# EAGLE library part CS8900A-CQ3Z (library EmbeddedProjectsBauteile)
Crystal LAN - Ethernet Controller
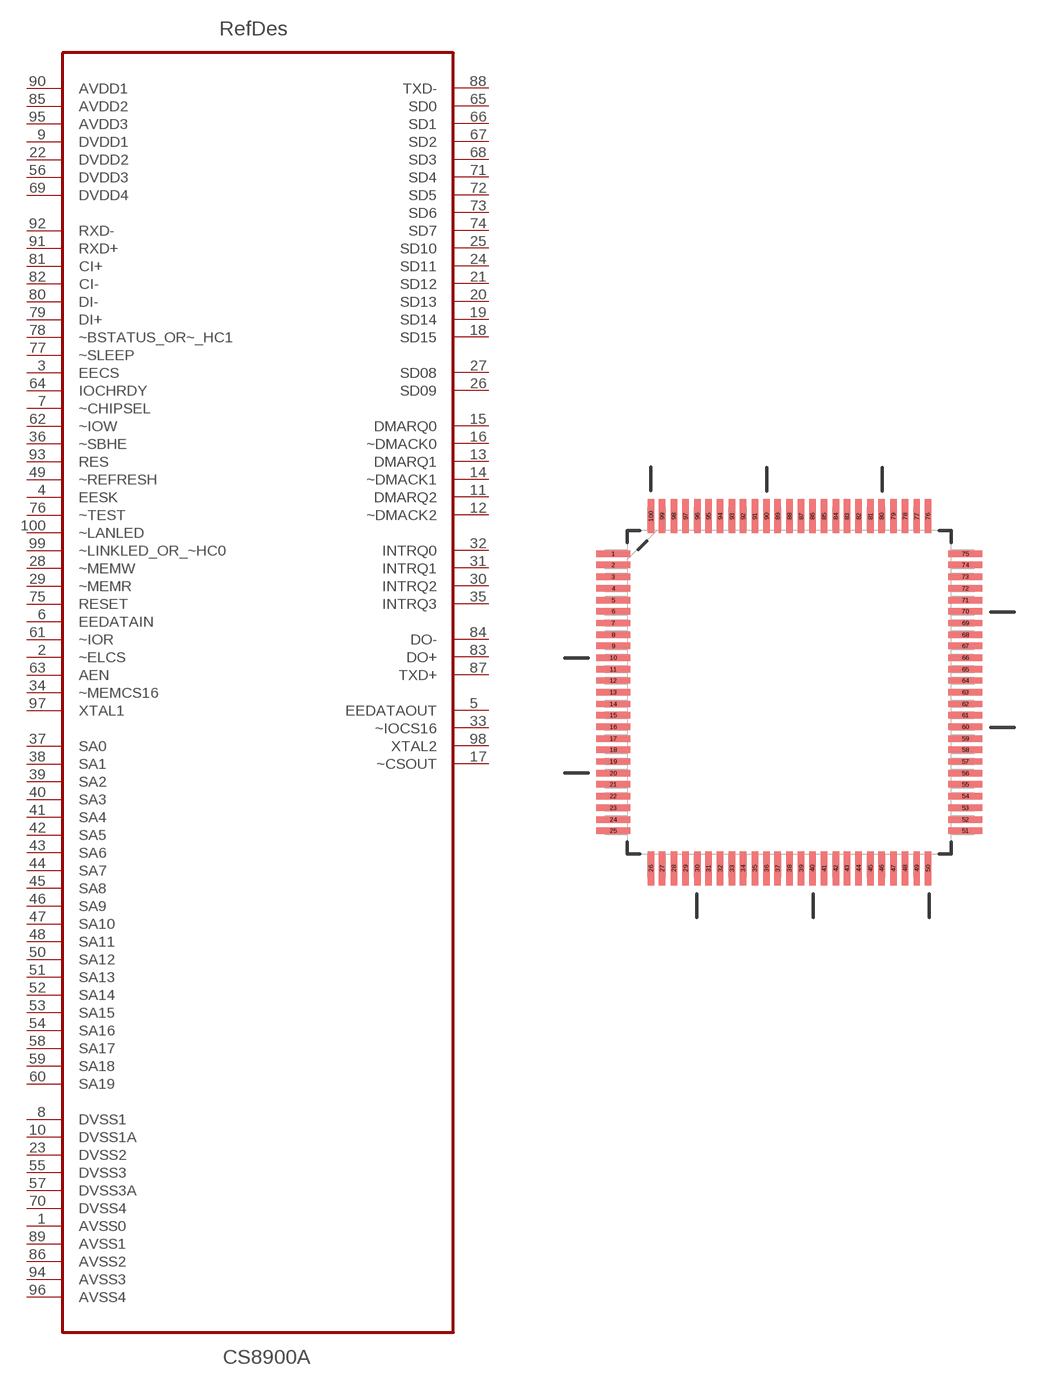
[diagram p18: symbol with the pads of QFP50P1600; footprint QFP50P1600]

Designator prefix IC

## CS8900A-CQ3Z (EP: 700081)  [QFP50P1600]
1  AVSS0  pwr
2  ~ELCS  in
3  EECS  in
4  EESK  in
5  EEDATAOUT  out
6  EEDATAIN  in
7  ~CHIPSEL  in
8  DVSS1  pwr
9  DVDD1  pwr
10  DVSS1A  pwr
11  DMARQ2  hiz
12  ~DMACK2  hiz
13  DMARQ1  hiz
14  ~DMACK1  hiz
15  DMARQ0  hiz
16  ~DMACK0  hiz
17  ~CSOUT  out
18  SD15  hiz
19  SD14  hiz
20  SD13  hiz
21  SD12  hiz
22  DVDD2  pwr
23  DVSS2  pwr
24  SD11  hiz
25  SD10  hiz
26  SD09  hiz
27  SD08  hiz
28  ~MEMW  in
29  ~MEMR  in
30  INTRQ2  out
31  INTRQ1  out
32  INTRQ0  out
33  ~IOCS16  out
34  ~MEMCS16  in
35  INTRQ3  out
36  ~SBHE  in
37  SA0  in
38  SA1  in
39  SA2  in
40  SA3  in
41  SA4  in
42  SA5  in
43  SA6  in
44  SA7  in
45  SA8  in
46  SA9  in
47  SA10  in
48  SA11  in
49  ~REFRESH  in
50  SA12  in
51  SA13  in
52  SA14  in
53  SA15  in
54  SA16  in
55  DVSS3  pwr
56  DVDD3  pwr
57  DVSS3A  pwr
58  SA17  in
59  SA18  in
60  SA19  in
61  ~IOR  in
62  ~IOW  in
63  AEN  in
64  IOCHRDY  in
65  SD0  hiz
66  SD1  hiz
67  SD2  hiz
68  SD3  hiz
69  DVDD4  pwr
70  DVSS4  pwr
71  SD4  hiz
72  SD5  hiz
73  SD6  hiz
74  SD7  hiz
75  RESET  in
76  ~TEST  in
77  ~SLEEP  in
78  ~BSTATUS_OR~_HC1  in
79  DI+  in
80  DI-  in
81  CI+  in
82  CI-  in
83  DO+  out
84  DO-  out
85  AVDD2  pwr
86  AVSS2  pwr
87  TXD+  out
88  TXD-  out
89  AVSS1  pwr
90  AVDD1  pwr
91  RXD+  in
92  RXD-  in
93  RES  in
94  AVSS3  pwr
95  AVDD3  pwr
96  AVSS4  pwr
97  XTAL1  in
98  XTAL2  out
99  ~LINKLED_OR_~HC0  pas
100  ~LANLED  pas

## Footprint QFP50P1600 (pad centres in mm)
smd 1.473 x 0.279: 1 -7.62,5.994; 2 -7.62,5.512; 3 -7.62,5.004; 4 -7.62,4.496; 5 -7.62,3.988; 6 -7.62,3.505; 7 -7.62,2.997; 8 -7.62,2.489; 9 -7.62,2.007; 10 -7.62,1.499; 11 -7.62,0.991; 12 -7.62,0.508; 13 -7.62,0; 14 -7.62,-0.508; 15 -7.62,-0.991; 16 -7.62,-1.499; 17 -7.62,-2.007; 18 -7.62,-2.489; 19 -7.62,-2.997; 20 -7.62,-3.505; 21 -7.62,-3.988; 22 -7.62,-4.496; 23 -7.62,-5.004; 24 -7.62,-5.512; 25 -7.62,-5.994; 51 7.62,-5.994; 52 7.62,-5.512; 53 7.62,-5.004; 54 7.62,-4.496; 55 7.62,-3.988; 56 7.62,-3.505; 57 7.62,-2.997; 58 7.62,-2.489; 59 7.62,-2.007; 60 7.62,-1.499; 61 7.62,-0.991; 62 7.62,-0.508; 63 7.62,0; 64 7.62,0.508; 65 7.62,0.991; 66 7.62,1.499; 67 7.62,2.007; 68 7.62,2.489; 69 7.62,2.997; 70 7.62,3.505; 71 7.62,3.988; 72 7.62,4.496; 73 7.62,5.004; 74 7.62,5.512; 75 7.62,5.994
smd 0.279 x 1.473: 26 -5.994,-7.62; 27 -5.512,-7.62; 28 -5.004,-7.62; 29 -4.496,-7.62; 30 -3.988,-7.62; 31 -3.505,-7.62; 32 -2.997,-7.62; 33 -2.489,-7.62; 34 -2.007,-7.62; 35 -1.499,-7.62; 36 -0.991,-7.62; 37 -0.508,-7.62; 38 0,-7.62; 39 0.508,-7.62; 40 0.991,-7.62; 41 1.499,-7.62; 42 2.007,-7.62; 43 2.489,-7.62; 44 2.997,-7.62; 45 3.505,-7.62; 46 3.988,-7.62; 47 4.496,-7.62; 48 5.004,-7.62; 49 5.512,-7.62; 50 5.994,-7.62; 76 5.994,7.62; 77 5.512,7.62; 78 5.004,7.62; 79 4.496,7.62; 80 3.988,7.62; 81 3.505,7.62; 82 2.997,7.62; 83 2.489,7.62; 84 2.007,7.62; 85 1.499,7.62; 86 0.991,7.62; 87 0.508,7.62; 88 0,7.62; 89 -0.508,7.62; 90 -0.991,7.62; 91 -1.499,7.62; 92 -2.007,7.62; 93 -2.489,7.62; 94 -2.997,7.62; 95 -3.505,7.62; 96 -3.988,7.62; 97 -4.496,7.62; 98 -5.004,7.62; 99 -5.512,7.62; 100 -5.994,7.62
